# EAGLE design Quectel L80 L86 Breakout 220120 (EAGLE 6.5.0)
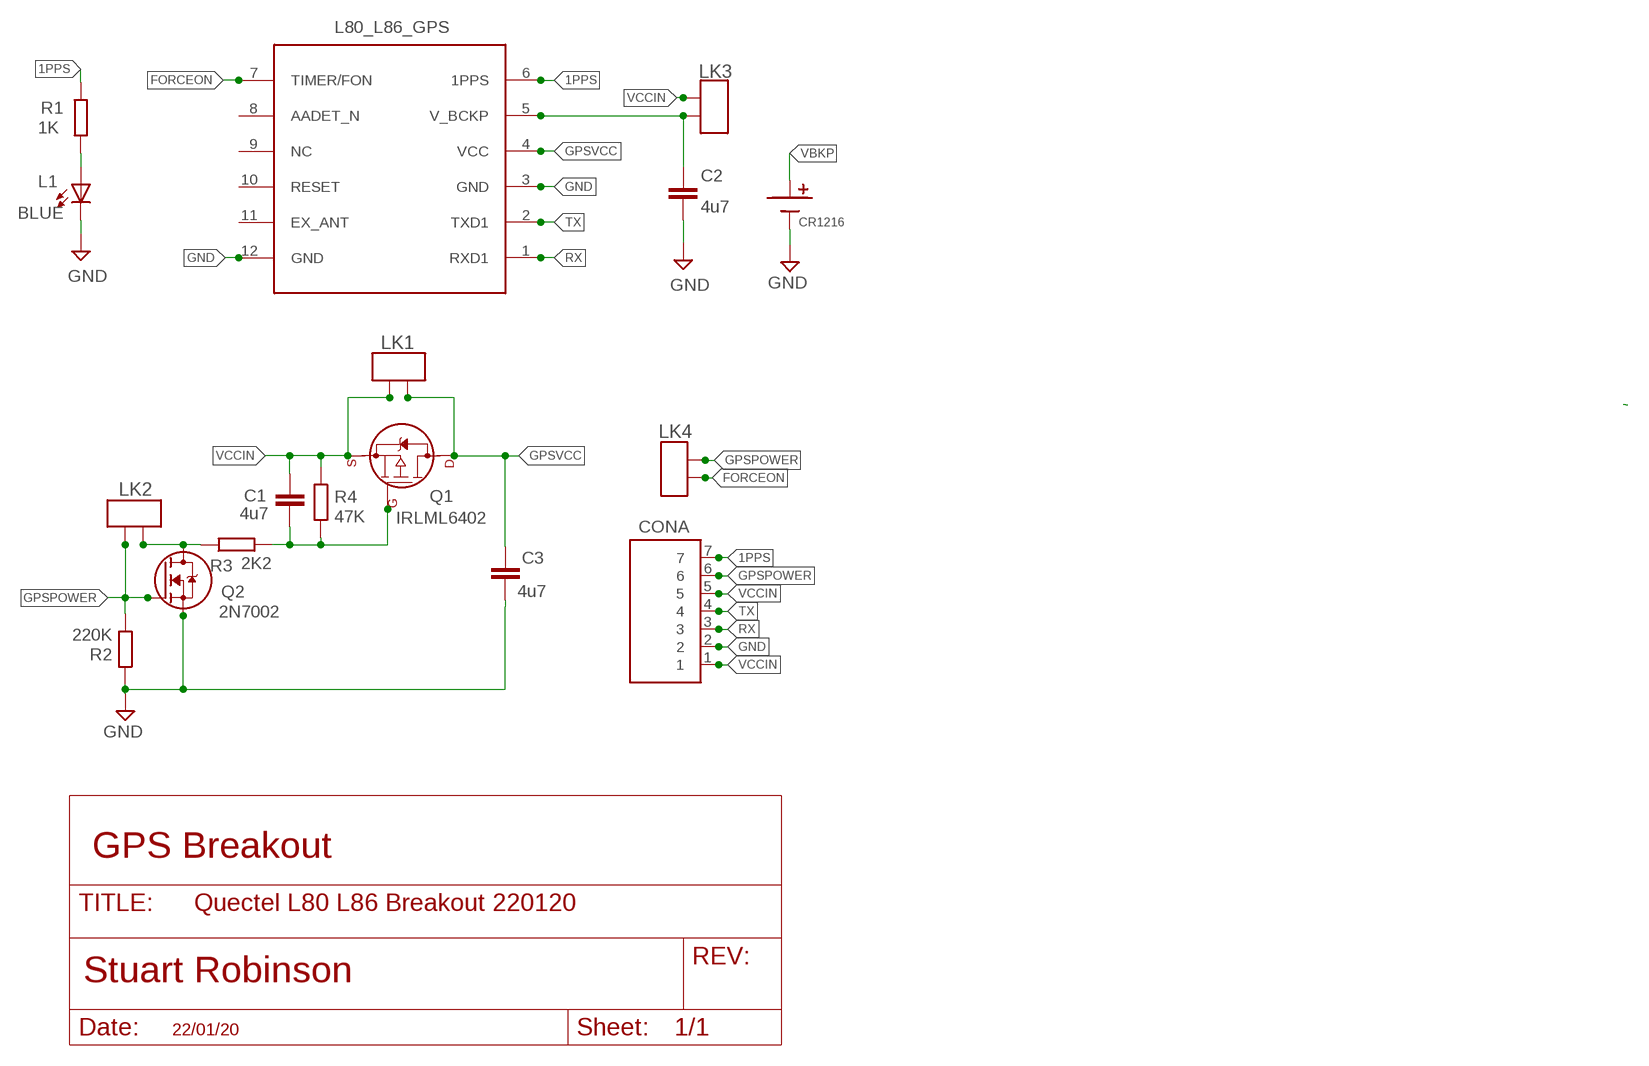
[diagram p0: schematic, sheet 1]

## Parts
BAT1  CR1216  12MMBATTERY  [12MMBATTERY]
C1  4u7  C805_REDUCED  [C0805_REDUCED]
C2  4u7  C805_REDUCED  [C0805_REDUCED]
C3  4u7  C805_REDUCED  [C0805_REDUCED]
CONA  7X1STD  [7X1]
L1  BLUE  0805LED  [0805LED]
L80_L86_GPS  L80_GNSS_MODULE  [L80_PACKAGE]
LK1  PCB_LINK_2  [PCB_LINK2]
LK2  PCB_LINK_2  [PCB_LINK2]
LK3  PCB_LINK_2  [PCB_LINK2]
LK4  PCB_LINK_2  [PCB_LINK2]
Q1  IRLML6402  IRLFL6402  [SOT23@1]
Q2  2N7002  NMOSFET  [SOT23]
R1  1K  R0805_REDUCED  [R0805_REDUCED]
R2  220K  R0805_REDUCED  [R0805_REDUCED]
R3  2K2  R0805_REDUCED  [R0805_REDUCED]
R4  47K  R0805_REDUCED  [R0805_REDUCED]

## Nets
1PPS: CONA.7 L80_L86_GPS.6(1PPS) R1.2
FORCEON: L80_L86_GPS.7(TIMER/FON) LK4.P$2
GND [GND]: BAT1.-VE(-) C2.2 C3.2 CONA.2 L1.C L80_L86_GPS.3(GND) L80_L86_GPS.12(GND) Q2.2(S) R2.1
GPSPOWER: CONA.6 LK2.P$1 LK4.P$1 Q2.1(G) R2.2
GPSVCC [VDD]: C3.1 L80_L86_GPS.4(VCC) LK1.P$1 Q1.3(D1)
N$2: C1.2 Q1.1(G1) R3.2 R4.2
N$3: LK2.P$2 Q2.3(D) R3.1
N$7: L1.A R1.1
RX: CONA.3 L80_L86_GPS.1(RXD1)
TX: CONA.4 L80_L86_GPS.2(TXD1)
VBKP: BAT1.+VE(+) C2.1 L80_L86_GPS.5(V_BCKP) LK3.P$2
VCCIN [VDD]: C1.1 CONA.1 CONA.5 LK1.P$2 LK3.P$1 Q1.2(S1) R4.1
Unconnected: L80_L86_GPS.8(AADET_N) L80_L86_GPS.9(NC) L80_L86_GPS.10(RESET) L80_L86_GPS.11(EX_ANT)

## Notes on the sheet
- GPS Breakout
- 22/01/20

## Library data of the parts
BAT1 = LMA2:12MMBATTERY
C1-C3 = resistor:C805_REDUCED
CONA = My_Pin_Headers:7X1
L1 = LMA2:0805LED
L80_L86_GPS = Quectel:L80_GNSS_MODULE: GPS module with an embedded patch antenna (15mmx15mmx4mm)
LK1-LK4 = LMA2:PCB_LINK_2
Q1 = LMA2:IRLFL6402
Q2 = LMA2:NMOSFET
R1-R4 = resistor:R0805_REDUCED

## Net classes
0 default: width 0.152 mm
1 GND: width 0.508 mm
2 VDD: width 0.508 mm
3 gpspower: width 0.508 mm

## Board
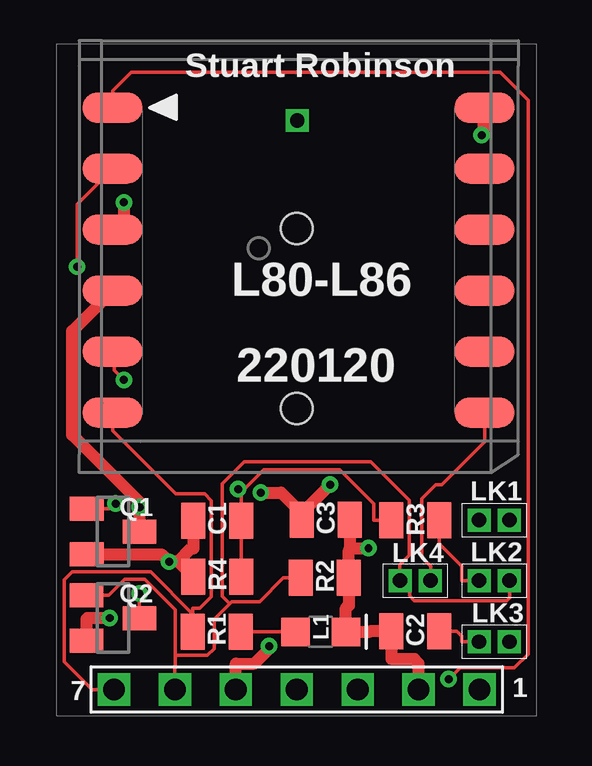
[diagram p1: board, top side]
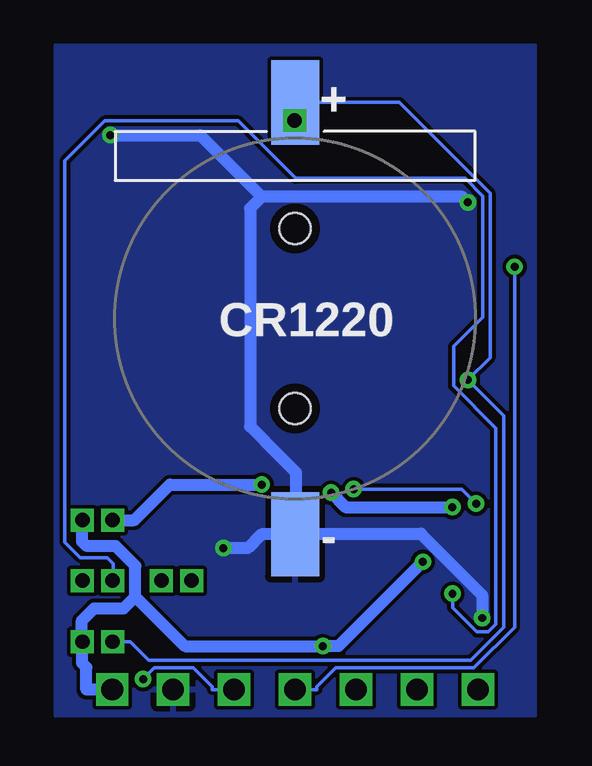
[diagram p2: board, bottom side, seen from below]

No outline drawn. Coordinates in mm, seen from the top.
Copper layers (1*16): Top 0.0356mm / dielectric 1.5011mm / Bottom 0.0356mm
Design rules "LaenPCBOrder *": minimum track width 6mil, minimum drill 13mil, track to track 6mil, track to pad 6mil, pad to pad 6mil, via to via 6mil, smd to smd 6mil, copper to edge 15mil, drill to drill 6mil, minimum pad ring 7mil, minimum via ring 7mil, stop-mask expansion 4mil, vias tented up to drill 1000mil, thermal gap 10mil
tRestrict: area 3.2,11.3 to 17.3,26.5

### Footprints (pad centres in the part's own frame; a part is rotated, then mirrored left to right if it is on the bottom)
12MMBATTERY = smd 3.54 x 2: +VE 9,0 | smd 3.5 x 2: -VE -9,0 | hole 1.3: -3.75,0; 3.75,0
C0805_REDUCED = smd 1 x 1.5: 1 -1,0; 2 1,0
7X1 = drill 0.9 square: 1 -7.62,0; 2 -5.08,0; 3 -2.54,0; 4 0,0; 5 2.54,0; 6 5.08,0; 7 7.62,0
0805LED = smd 1.2 x 1.2: A 0,-1.05; C 0,1.05
L80_PACKAGE = smd 2.5 x 1.25: 1 15.75,1.8; 2 15.75,4.34; 3 15.75,6.88; 4 15.75,9.42; 5 15.75,11.96; 6 15.75,14.5; 7 0.25,14.5; 8 0.25,11.96; 9 0.25,9.42; 10 0.25,6.88; 11 0.25,4.34; 12 0.25,1.8
PCB_LINK2 = drill 0.6 square: P$1 -0.63,0; P$2 0.63,0
SOT23@1 = smd 1 x 1.4: 1 -0.95,-1.1; 2 0.95,-1.1; 3 0,1.1
SOT23 = smd 1 x 1.4: 1 -0.95,-1.1; 2 0.95,-1.1; 3 0,1.1
R0805_REDUCED = smd 1 x 1.5: 1 -1,0; 2 1,0

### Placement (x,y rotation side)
BAT1  10,16.56 90 bottom
C1  6.69,8.14 0 top
C2  14.94,3.52 180 top
C3  11.21,8.18 0 top
CONA  10,1.1 180 top
L1  11,3.5 270 top
L80_L86_GPS  18.08,27.14 180 top
LK1  18.23,8.16 0 top
LK2  18.23,5.64 180 top
LK3  18.23,3.09 180 top
LK4  14.94,5.64 0 top
Q1  2.35,7.68 270 top
Q2  2.34,4.08 270 top
R1  6.67,3.5 180 top
R2  11.17,5.75 180 top
R3  14.94,8.15 180 top
R4  6.69,5.79 0 top

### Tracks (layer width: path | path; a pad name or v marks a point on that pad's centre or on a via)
1PPS
  Top 0.152: CONA.7 1.48,1.1 0.31,2.27 0.31,5.67 0.64,6 3.91,6 5.67,4.23 | 5.67,4.23 5.67,4.48 5.96,4.48 6.44,4.96 6.44,8.97 6.16,9.25 4.95,9.25 2.33,11.87 L80_L86_GPS.6 | R1.2 5.67,4.23
FORCEON
  Top 0.152: LK4.P$2 15.59,6.24 15.21,6.62 15.21,9.05 15.79,9.63 16.04,9.63 17.83,11.41 L80_L86_GPS.7
GND  (via drill 0.33 pad 0.69)
  Top 0.508: 12.21,6.99 v12.99,6.99 | 12.21,6.99 12.21,6.95 12.17,6.91 R2.1 12.17,4.59 12.14,4.59 12.05,4.51 L1.C 13.01,3.5 13.03,3.52 C2.2 13.94,2.36 14.9,2.36 15.08,2.18 CONA.2 | 12.21,6.99 12.21,7.17 C3.2 | Q2.2 1.24,4.04 1.28,4.08 v2.21,4.08 | v17.7,24.2 17.8,24.3 17.8,25.3 L80_L86_GPS.12 | v2.8,21.4 2.8,20.73 L80_L86_GPS.3
  Bottom 0.508: 9.97,7.59 4.76,7.59 2.21,5.04 v2.21,4.08 | v12.99,6.99 11.97,6.99 11.41,7.56 BAT1.-VE 9.97,7.59 | 9.97,7.59 9.97,10.14 11.23,11.4 11.23,11.42 11.87,12.06 11.87,21.15 11.39,21.63 | v2.8,21.4 2.88,21.48 3.03,21.63 11.39,21.63 | v17.7,24.2 13.96,24.2 11.39,21.63
  pour Bottom: 0,27.94 20,27.94 20,0 0,0
GPSPOWER
  Top 0.152: 7.21,4.68 6.56,4.03 6.56,2.79 6.28,2.52 4.94,2.52 | 7.21,4.68 7.29,4.76 8.45,4.76 9.44,5.75 R2.2 | 7.21,4.68 6.91,4.99 6.91,9.67 7.82,10.58 13.09,10.58 14.69,8.98 14.69,6.8 14.69,6.69 14.29,6.29 14.29,5.66 LK4.P$1 14.7,5.25 14.7,5 14.9,4.8 18.75,4.8 18.88,4.93 LK2.P$1 | 4.94,2.52 4.94,2.02 4.92,2 CONA.6 | 4.94,2.52 4.94,4.42 3.67,5.69 2.83,5.69 2.17,5.03 Q2.1
GPSVCC  (via drill 0.33 pad 0.69)
  Top 0.508: L80_L86_GPS.4 0.64,16.03 0.64,11.71 3.45,8.91 v3.45,8.7 3.45,8.32 Q1.3 | 10.2,8.45 v11.39,9.64 | 10.2,8.45 10.2,8.2 C3.1 | v8.5,9.3 9.35,9.3 10.2,8.45
  Bottom 0.508: v11.39,9.64 15.22,9.64 16.7,8.16 LK1.P$1 | v8.5,9.3 7.9,8.7 v3.45,8.7
N$2  (via drill 0.33 pad 0.69)
  Top 0.152: 7.69,9.32 v7.56,9.45 | 7.69,9.32 8.62,10.26 11.79,10.26 13.21,8.83 13.21,8.15 R3.2 | 7.69,9.32 7.69,9.12 C1.2 R4.2 | Q1.1 2.18,8.63 2.39,8.85 v2.45,8.85
  Bottom 0.152: v2.45,8.85 3.06,9.45 v7.56,9.45
N$3  (via drill 0.33 pad 0.69)
  Top 0.152: LK2.P$2 16.87,5.64 16.87,6.24 15.94,7.17 R3.1 | Q2.3 v3.44,5.09
  Bottom 0.152: v3.44,5.09 3.44,4.5 2.44,3.5 1.95,3.5 1.63,3.81 1.63,11.99 3.39,13.75 3.39,15.4 2.18,16.61 2.18,21.66 2.92,22.39 9.97,22.39 12.37,24.79 17.94,24.79 19.6,23.13 19.6,7.24 18.94,6.59 17.82,6.59 17.58,6.35 LK2.P$2
N$7
  Top 0.152: R1.1 L1.A
RX  (via drill 0.33 pad 0.69)
  Top 0.152: L80_L86_GPS.1 2.33,26.05 3.1,26.82 18.47,26.82 19.64,25.65 19.64,2.57 19.07,2 16.8,2 v16.33,1.53
  Bottom 0.152: v16.33,1.53 15.86,2 14.23,2 13.44,1.21 13.44,1.1 CONA.3
S$1  (via drill 0.6)
  other vias: 10.02,24.81
TX  (via drill 0.33 pad 0.69)
  Top 0.152: L80_L86_GPS.2 0.85,21.32 v0.85,18.71
  Bottom 0.152: v0.85,18.71 0.85,3.7 2.55,2 8.31,2 9.1,1.21 9.1,1.1 CONA.4
VBKP  (via drill 0.33 pad 0.69)
  Top 0.152: LK3.P$2 16.87,3.09 16.87,3.31 16.67,3.52 C2.1 | v2.8,14 2.4,14.4 2.4,15.1 L80_L86_GPS.5
  Bottom 0.152: LK3.P$2 16.87,3.09 16.11,2.32 2.69,2.32 1.31,3.7 1.31,12.51 v2.8,14 1.87,14.93 1.87,21.78 5.65,25.56 BAT1.+VE
VCCIN  (via drill 0.33 pad 0.69)
  Top 0.508: C1.1 5.69,6.98 5.61,6.98 5.05,6.42 | 5.05,6.42 v4.68,6.42 4.37,6.73 Q1.2 | R4.1 5.05,6.42 | CONA.5 7.46,2.18 8.22,2.18 8.85,2.81 v8.85,2.91
  Bottom 0.508: v4.68,6.42 8.19,2.91 v8.85,2.91 14.6,2.91 16.66,4.97 | 16.66,4.97 16.66,6.25 17.48,7.07 18.68,7.07 18.88,7.28 LK1.P$2 | 16.66,4.97 17.14,4.48 18.37,4.48 18.88,3.97 LK3.P$1 18.88,2.65 18.88,2.21 18.7,2.03 18.7,1.1 CONA.1

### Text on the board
tNames: Stuart Robinson | L80-L86 | 220120 | Q1 | C1 | C3 | LK1 | R3 | R4 | R2 | LK4 | LK2 | Q2 | R1 | L1 | LK3 | C2 | 7 | 1
bNames: + | CR1220 | -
